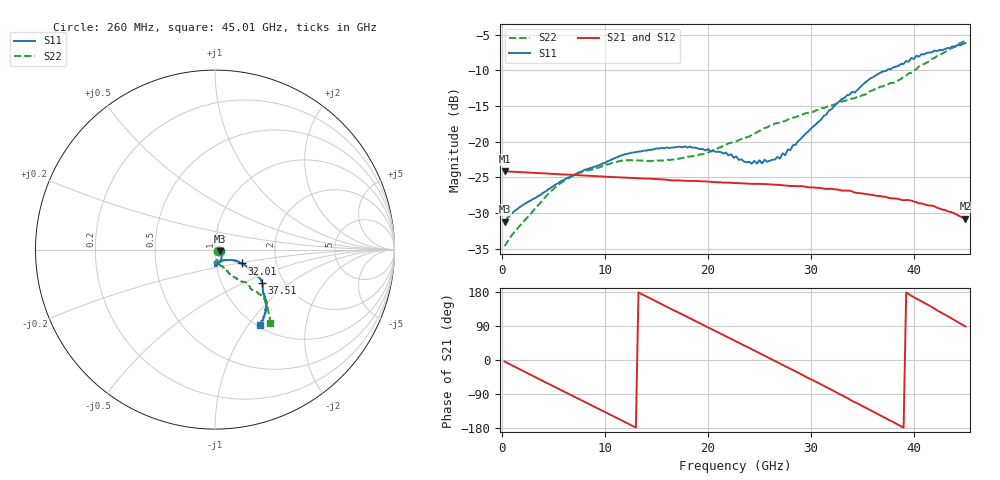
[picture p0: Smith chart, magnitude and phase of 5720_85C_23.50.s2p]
! Device:  ADRF5720
! Description: 0.5dB LSB GaAs MMIC 6-bit Digital Attenuator
! Frequency:  0.000009 -  40 GHz
! Ports:
!	RF1	= Port 1
!	RF2	= Port 2
! Vdd:  3.3 Volt
! Vss:  -3.3 Volt
! Control:  0/3.3 Volt
! State:  23.50 dB attenuation
! Data:  The device was measured using G-S-G Probes on a matrix board.
!  Data was collected using an calibrated 4 port network analyzer.
!  The reference plane for this measurement is at the launchers.
! Note:  Analog Devices supplies this data as a sample of measured data
!  for this product.  Your particular data for this product may vary.
!  Data was taken at 85 degrees C.
!  Analog Devices reserves the right to change this data at anytime.
# GHZ S DB R 45.0
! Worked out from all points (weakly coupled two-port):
!   180 points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, 260 MHz to 45.01 GHz, reference 45 ohm
!   highest |S21| = -24.13 dB at 260 MHz (marker M1); lowest = -30.8 dB at 45.01 GHz (marker M2)
!   lowest |S11| = -31.2 dB at 260 MHz (marker M3), VSWR 1.06, Z = 47.4 - j0.763 ohm
!   |S11| at or under -10 dB: start of sweep to 37.37 GHz
!   |S22| runs from -34.6 to -5.8 dB; largest |S21 - S12| = 0.00037
!   S11 on the Smith chart (normalised r, x): 260 MHz: 1.05, -0.02; 32.01 GHz: 1.33, -0.21; 37.51 GHz: 1.55, -0.64; 45.01 GHz: 1.02, -1.14
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0.26  -31.16 -16.9  -24.13 -3.8  -24.12 -3.8  -34.61 -26.0
1.26  -29.64 -3.6  -24.22 -18.0  -24.21 -17.9  -32.51 -13.7
4.76  -26.43 -38.3  -24.48 -66.0  -24.46 -66.0  -26.93 -65.2
7.76  -24.16 -55.8  -24.71 -106.8  -24.70 -106.8  -24.25 -81.5
11.51  -21.96 -73.5  -24.99 -157.8  -24.98 -157.7  -22.67 -92.4
15.26  -20.95 -84.7  -25.24 150.7  -25.22 150.9  -22.63 -90.7
18.26  -20.68 -90.0  -25.48 110.1  -25.46 110.3  -22.05 -82.2
22.76  -22.05 -83.9  -25.78 48.7  -25.77 48.9  -19.91 -67.5
24.26  -23.07 -75.8  -25.89 28.4  -25.87 28.6  -19.05 -64.4
27.01  -22.36 -49.8  -26.04 -9.6  -26.02 -9.3  -17.29 -60.0
27.26  -21.61 -46.0  -26.09 -13.1  -26.08 -12.8  -17.17 -60.4
27.51  -21.89 -45.2  -26.13 -16.4  -26.12 -16.1  -17.10 -59.4
27.76  -21.08 -41.6  -26.15 -19.8  -26.13 -19.5  -16.88 -60.2
28.01  -21.19 -42.0  -26.19 -23.2  -26.18 -22.9  -16.81 -59.6
30.26  -17.84 -30.1  -26.40 -54.2  -26.38 -54.0  -15.81 -58.5
32.01  -15.46 -27.1  -26.59 -78.6  -26.58 -78.3  -14.92 -56.5
35.76  -11.16 -31.7  -27.40 -132.1  -27.39 -131.8  -12.93 -51.1
37.51  -9.84 -35.2  -27.84 -157.2  -27.82 -156.8  -11.94 -46.5
37.76  -9.85 -35.5  -27.91 -160.6  -27.88 -160.2  -11.77 -46.7
41.51  -7.53 -47.3  -28.94 143.5  -28.93 144.0  -8.73 -44.4
43.51  -6.90 -51.5  -29.80 112.5  -29.77 112.9  -6.98 -48.7
45.01  -6.21 -59.5  -30.78 88.7  -30.77 88.9  -5.83 -53.2
